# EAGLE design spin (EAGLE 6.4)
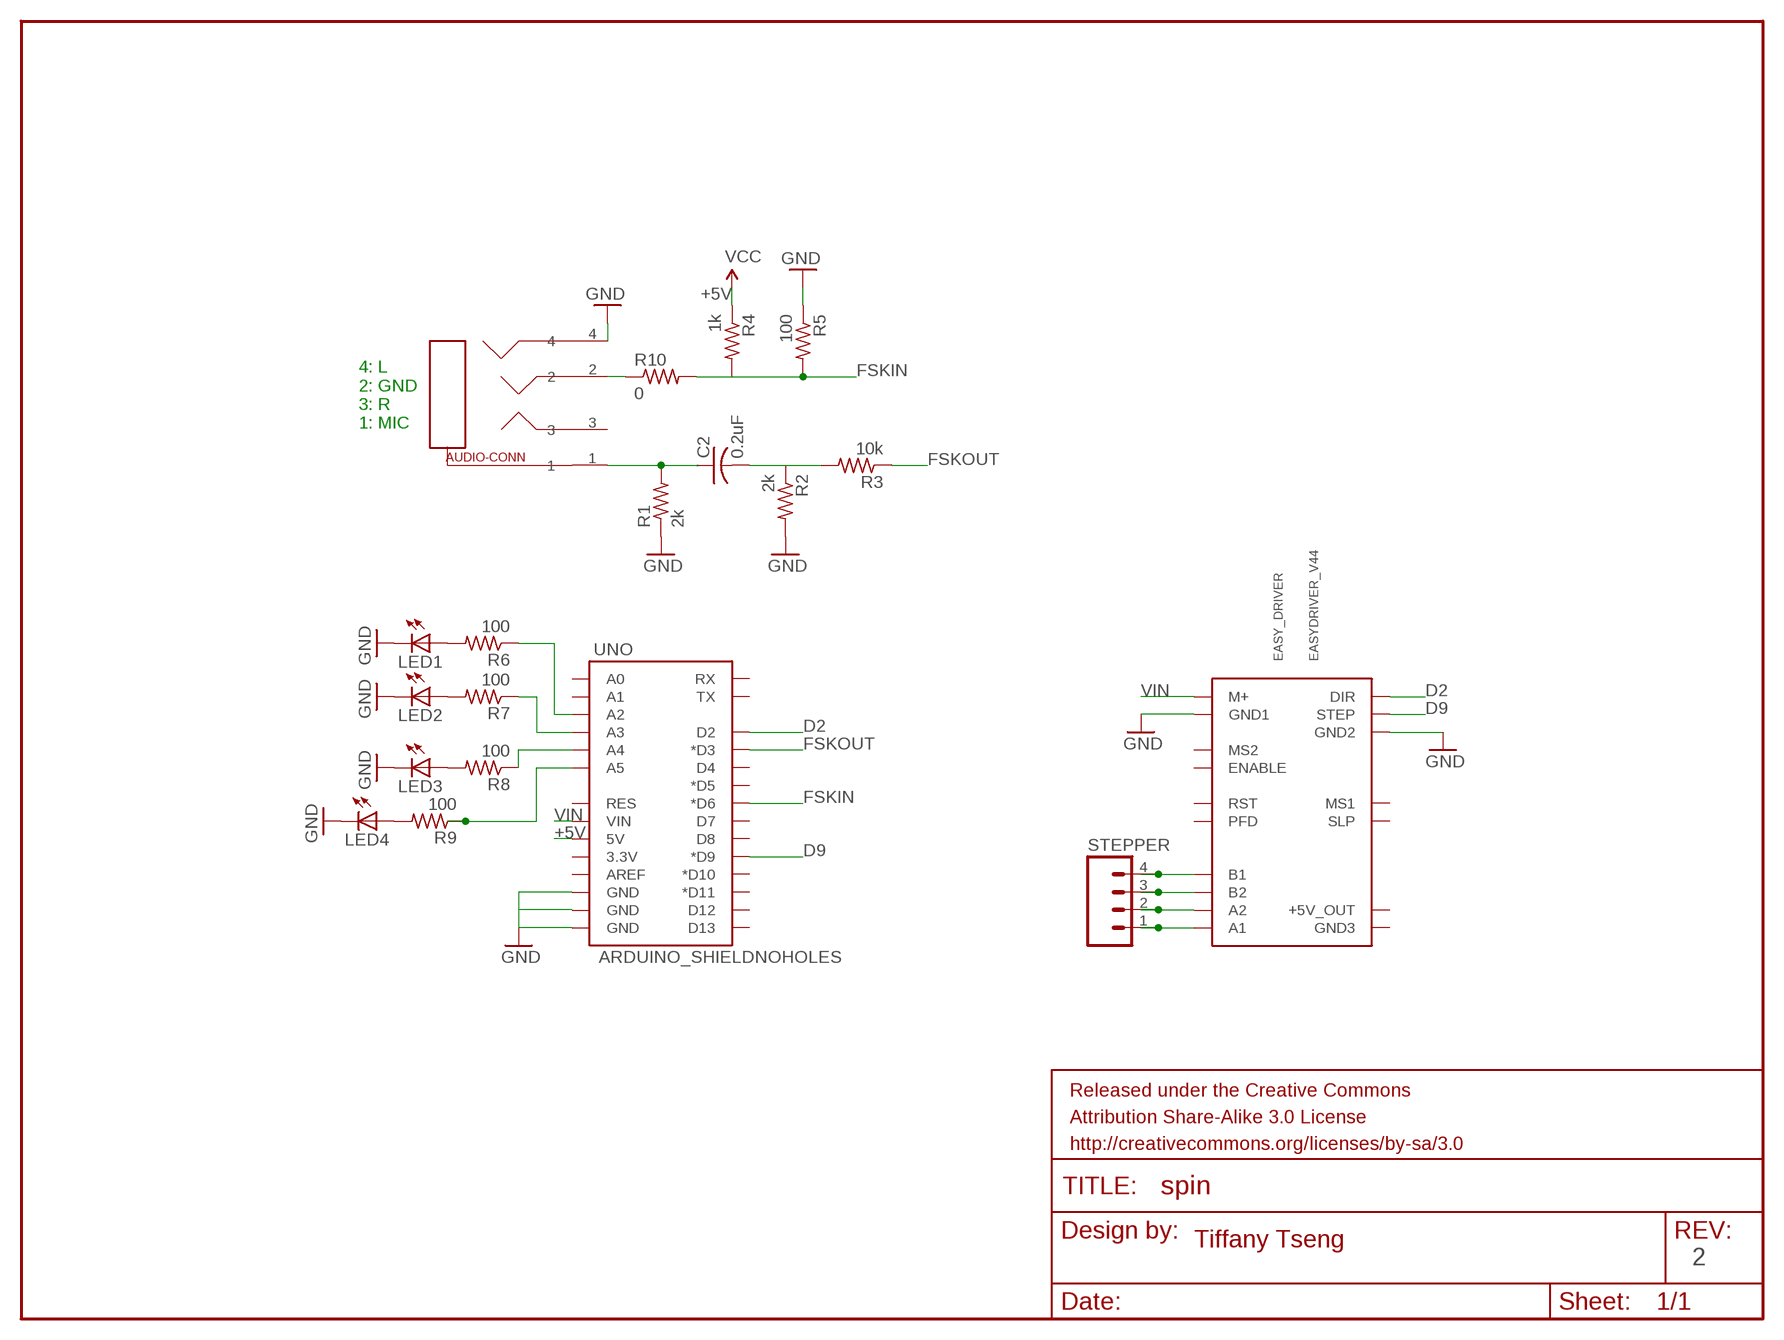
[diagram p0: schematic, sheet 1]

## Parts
C2  0.2uF  C-USC1206  [C1206]
EASY_DRIVER  EASYDRIVER_V44  [EASYDRIVER_V44]
FRAME1  FRAME-LETTER  [CREATIVE_COMMONS]
LED1  LED1206  [1206]
LED2  LED1206  [1206]
LED3  LED1206  [1206]
LED4  LED1206  [1206]
R1  2k  R-US_R1206  [R1206]
R2  2k  R-US_R1206  [R1206]
R3  10k  R-US_R1206  [R1206]
R4  1k  R-US_R1206  [R1206]
R5  100  R-US_R1206  [R1206]
R6  100  R-US_R1206  [R1206]
R7  100  R-US_R1206  [R1206]
R8  100  R-US_R1206  [R1206]
R9  100  R-US_R1206  [R1206]
R10  0  R-US_R1206  [R1206]
STEPPER  M04PTH  [1X04]
U$1  SJ-43514  [SJ-43514]
UNO  ARDUINO_SHIELDNOHOLES  [DUEMILANOVE_SHIELD_NOHOLES]

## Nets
1: C2.1 R1.2 U$1.1
2: R10.1 U$1.2
+5V: R4.1 UNO.5V ; supply symbol labelled VCC
D2: EASY_DRIVER.DIR UNO.D2
D9: EASY_DRIVER.STEP UNO.D9(*D9)
FSKIN: R4.2 R5.2 R10.2 UNO.D6(*D6)
FSKOUT: R3.1 UNO.D3(*D3)
GND: EASY_DRIVER.GND1 EASY_DRIVER.GND2 LED1.2(C) LED2.2(C) LED3.2(C) LED4.2(C) R1.1 R2.2 R5.1 U$1.4 UNO.GND@0(GND) UNO.GND@1(GND) UNO.GND@2(GND)
N$2: C2.2 R2.1 R3.2
N$4: EASY_DRIVER.B1 STEPPER.4
N$5: EASY_DRIVER.B2 STEPPER.3
N$6: EASY_DRIVER.A2 STEPPER.2
N$7: EASY_DRIVER.A1 STEPPER.1
N$10: R9.1 UNO.A5
N$11: LED1.1(A) R6.2
N$12: LED2.1(A) R7.2
N$13: R8.1 UNO.A4
N$14: LED3.1(A) R8.2
N$15: R7.1 UNO.A3
N$16: LED4.1(A) R9.2
N$17: R6.1 UNO.A2
VIN: EASY_DRIVER.M+ UNO.VIN
Unconnected: EASY_DRIVER.ENABLE EASY_DRIVER.GND3 EASY_DRIVER.MS1 EASY_DRIVER.MS2 EASY_DRIVER.P$11(+5V_OUT) EASY_DRIVER.PFD EASY_DRIVER.RST EASY_DRIVER.SLEEP(SLP) U$1.3 UNO.3.3V UNO.A0 UNO.A1 UNO.AREF UNO.D4 UNO.D5(*D5) UNO.D7 UNO.D8 UNO.D10(*D10) UNO.D11(*D11) UNO.D12 UNO.D13 UNO.RES UNO.RX UNO.TX

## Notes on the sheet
- 4: L
  2: GND
  3: R
  1: MIC
- Tiffany Tseng
- 2

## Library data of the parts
C2 = rcl:C-US: CAPACITOR, American symbol
EASY_DRIVER = EasyDriver:EASYDRIVER_V44: EasyDriver version 4.4 - http://www.schmalzhaus.com/EasyDriver
FRAME1 = SparkFun-Aesthetics:FRAME-LETTER: Schematic Frame
LED1-LED4 = ng:LED
R1-R10 = rcl:R-US_: RESISTOR, American symbol
STEPPER = SparkFun-Connectors:M04: Header 4 Standard 4-pin 0.1" header. Use with straight break away headers (SKU : PRT-00116), right angle break away headers (PRT-00553), swiss pins (PRT-00743), machine pins (PRT-00117), and female headers (PRT-00115). Molex polarized connector foot print use with SKU : PRT-08231 with associated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
U$1 = spin:SJ-43514
UNO = SparkFun-Boards:ARDUINO_SHIELD: Arduino shield footprint

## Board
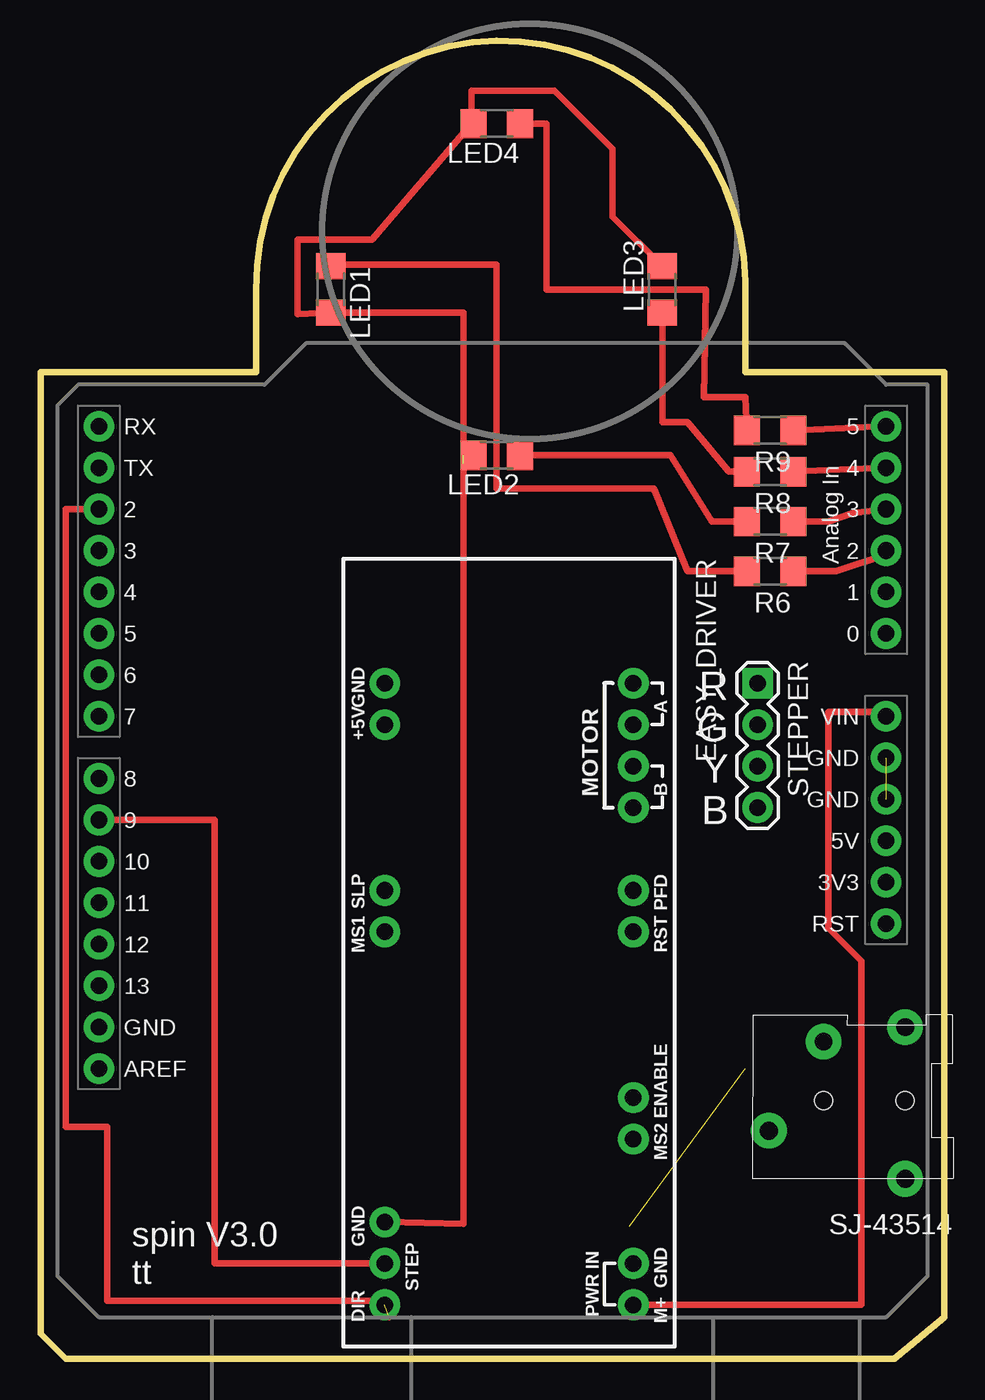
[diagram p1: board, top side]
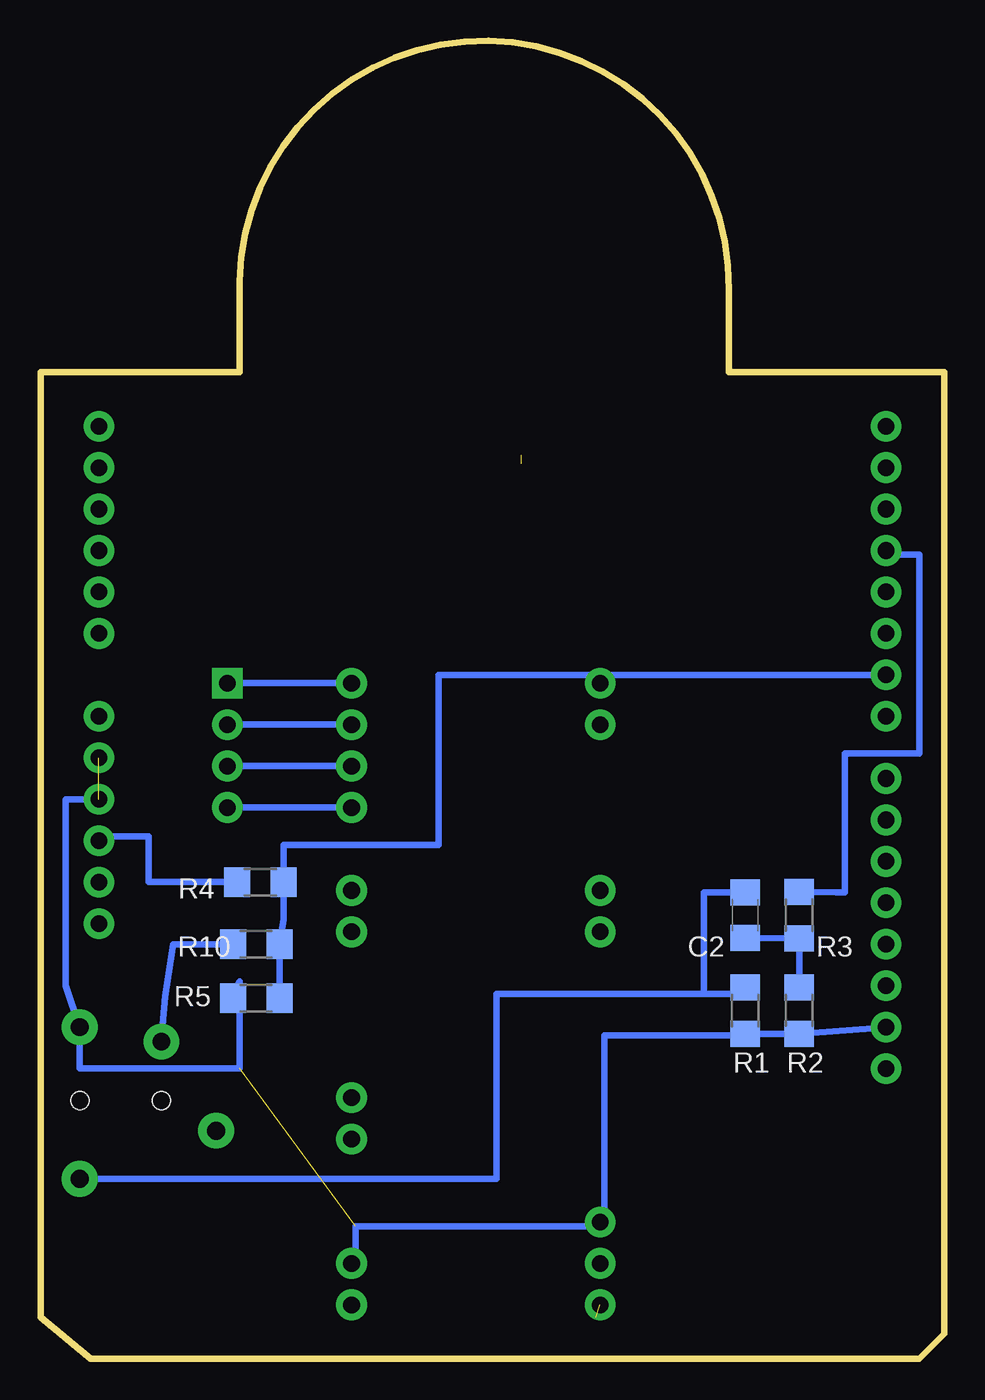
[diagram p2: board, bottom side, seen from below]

Size 55.37 x 80.77 mm. Coordinates in mm from the lower left corner, seen from the top.
Outline: 55.37,55.88 55.37,2.54 52.32,0 3.56,0 1.52,0 0,1.52 0,55.37 0,60.45 13.21,60.45 13.21,65.53 arc-180 43.18,66.04 43.18,60.45 55.37,60.45 55.37,55.88
Copper layers (1*16): Top 0.035mm / dielectric 1.5mm / Bottom 0.035mm
Design rules "default": minimum track width 10mil, minimum drill 24mil, track to track 8mil, track to pad 8mil, pad to pad 8mil, via to via 8mil, smd to smd 8mil, copper to edge 40mil, drill to drill 8mil, minimum pad ring 10mil, minimum via ring 8mil, stop-mask expansion 4mil, vias tented up to drill 0mil, thermal gap 10mil

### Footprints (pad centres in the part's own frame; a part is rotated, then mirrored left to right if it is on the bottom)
C1206 = smd 1.6 x 1.8: 1 -1.4,0; 2 1.4,0
EASYDRIVER_V44 = drill 1.016 pad 1.88: A1 -16.51,7.62; A2 -13.97,7.62; B1 -8.89,7.62; B2 -11.43,7.62; DIR 21.59,-7.62; ENABLE 8.89,7.62; GND1 19.05,7.62; GND2 16.51,-7.62; GND3 -16.51,-7.62; M+ 21.59,7.62; MS1 -1.27,-7.62; MS2 11.43,7.62; P$11 -13.97,-7.62; PFD -3.81,7.62; RST -1.27,7.62; SLEEP -3.81,-7.62; STEP 19.05,-7.62
1206 = smd 1.6 x 1.803: 1 -1.422,0; 2 1.422,0
R1206 = smd 1.6 x 1.803: 1 -1.422,0; 2 1.422,0
1X04 = drill 1.016 pad 1.88 square: 1 0,0 | drill 1.016 pad 1.88: 2 2.54,0; 3 5.08,0; 4 7.62,0
SJ-43514 = drill 1.092 pad 2.184: 1 2.896,9.296; 2 7.899,0.889; 3 11.252,6.35; 4 2.896,0 | hole 1.092: 2.896,4.496; 7.899,4.496
DUEMILANOVE_SHIELD_NOHOLES = drill 1.016 pad 1.88: 3.3V 50.8,26.67; 5V 50.8,29.21; A0 50.8,41.91; A1 50.8,44.45; A2 50.8,46.99; A3 50.8,49.53; A4 50.8,52.07; A5 50.8,54.61; AREF 2.54,15.24; D2 2.54,49.53; D3 2.54,46.99; D4 2.54,44.45; D5 2.54,41.91; D6 2.54,39.37; D7 2.54,36.83; D8 2.54,33.02; D9 2.54,30.48; D10 2.54,27.94; D11 2.54,25.4; D12 2.54,22.86; D13 2.54,20.32; GND@0 50.8,31.75; GND@1 50.8,34.29; GND@2 2.54,17.78; RES 50.8,24.13; RX 2.54,54.61; TX 2.54,52.07; VIN 50.8,36.83

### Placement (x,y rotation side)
C2  12.19,27.18 270 bottom
EASY_DRIVER  28.7,24.89 270 top
FRAME1  not placed on the board
LED1  17.78,65.53 270 top
LED2  27.94,55.37 180 top
LED3  38.1,65.53 90 top
LED4  27.94,75.69 180 top
R1  12.19,21.34 90 bottom
R2  8.89,21.34 270 bottom
R3  8.89,27.18 270 bottom
R4  41.91,29.21 0 bottom
R5  42.16,22.1 0 bottom
R6  44.7,48.26 180 top
R7  44.7,51.31 180 top
R8  44.7,54.36 180 top
R9  44.7,56.9 180 top
R10  42.16,25.4 0 bottom
STEPPER  43.94,41.4 270 top
U$1  55.88,20.32 180 top
UNO  1.02,2.54 0 top

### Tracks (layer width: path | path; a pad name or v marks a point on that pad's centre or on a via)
1
  Bottom 0.406: C2.1 14.73,28.58 14.73,22.35 | 14.73,22.35 12.19,22.35 | 12.19,22.35 R1.2 12.19,22.35 | U$1.1 27.43,11.02 27.43,22.35 14.73,22.35 | 14.73,22.35 12.19,22.35
2
  Bottom 0.406: R10.1 45.72,25.4 47.24,25.4 47.75,22.2 U$1.2
+5V
  Bottom 0.406: R4.1 48.77,29.21 48.77,32 51.82,32 UNO.5V
D2  (1 unrouted)
  Top 0.406: UNO.D2 1.52,52.07 1.52,14.22 4.06,14.22 4.06,3.56 21.34,3.56 21.34,2.54
D9
  Top 0.406: EASY_DRIVER.STEP 10.67,5.84 10.67,33.02 UNO.D9
FSKIN
  Bottom 0.406: R5.2 R10.2 40.49,26.92 R4.2 40.49,31.5 30.99,31.5 30.99,41.91 UNO.D6
FSKOUT
  Bottom 0.406: R3.1 6.6,28.58 6.1,28.58 6.1,37.08 1.52,37.08 1.52,49.28 3.56,49.28 UNO.D3
GND  (3 unrouted)
  Top 0.406: LED4.2 26.42,75.69 | 26.42,75.69 26.42,77.72 31.5,77.72 35.05,74.17 35.05,70 LED3.2 | 26.42,75.69 20.32,68.58 15.75,68.58 15.75,64.01 LED1.2 25.91,64.11 25.91,54.86 | LED2.2 25.91,55.37 25.91,8.28 EASY_DRIVER.GND2
  Bottom 0.406: UNO.GND@2 R2.2 11.68,19.91 | 11.68,19.91 R1.1 | 11.68,19.91 11.68,19.81 20.83,19.81 20.83,8.13 21.34,8.13 21.34,8.38 EASY_DRIVER.GND2 21.08,8.13 36.07,8.13 36.07,5.84 EASY_DRIVER.GND1 | R5.1 43.18,23.11 43.18,17.78 45.21,17.78 52.98,17.78 U$1.4 53.85,22.86 53.85,34.29 UNO.GND@0
N$2
  Bottom 0.406: C2.2 R3.2 R2.1
N$4
  Bottom 0.406: EASY_DRIVER.B1 STEPPER.4
N$5
  Bottom 0.406: EASY_DRIVER.B2 STEPPER.3
N$6
  Bottom 0.406: EASY_DRIVER.A2 STEPPER.2
N$7
  Bottom 0.406: EASY_DRIVER.A1 STEPPER.1
N$10
  Top 0.406: R9.1 UNO.A5
N$11
  Top 0.406: LED1.1 17.78,67.06 23.88,67.06 27.94,67.06 27.94,53.34 37.59,53.34 39.62,48.26 R6.2
N$12
  Top 0.406: LED2.1 38.61,55.37 41.15,51.31 R7.2
N$13
  Top 0.406: R8.1 UNO.A4
N$14
  Top 0.406: R8.2 42.16,54.36 39.62,57.4 38.1,57.4 LED3.1
N$15
  Top 0.406: R7.1 48.26,51.31 49.78,51.82 UNO.A3
N$16
  Top 0.406: LED4.1 30.99,75.69 30.99,65.53 40.76,65.53 40.64,58.93 43.18,58.93 R9.2
N$17
  Top 0.406: R6.1 48.77,48.26 51.82,49.28 UNO.A2
VIN
  Top 0.406: EASY_DRIVER.M+ 50.29,3.3 50.29,24.38 48.26,26.42 48.26,39.62 51.82,39.62 UNO.VIN

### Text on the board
tPlace: spin V3.0 / tt
tNames: R | G | Y | B

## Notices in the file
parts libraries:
SparkFun-Connectors: Licensing: CC v3.0 Share-Alike You are welcome to use this library for commercial purposes.
SparkFun-Aesthetics: Released under the Creative Commons Attribution Share-Alike 3.0 License
SparkFun-Aesthetics: http://creativecommons.org/licenses/by-sa/3.0
